DATA_BLOCK DB 99
NAME : OhneName
VERSION : 1.0


 STRUCT
  OFFSET_TABLE: STRUCT
   Offset_Table : STRUCT
    Offset_Type : WORD := W#16#1;
    Offset_Length : WORD := W#16#1E;
    Offset_Address : WORD := W#16#0;
   END_STRUCT ;
   Processdata_Long_Table : STRUCT
    Processdata_Long_Type : WORD := W#16#6;
    Processdata_Long_Length : WORD := W#16#C;
    Processdata_Long_Address : WORD := W#16#1E;
   END_STRUCT ;
   Control_Table : STRUCT
    Control_Type : WORD := W#16#5;
    Control_Length : WORD := W#16#6;
    Control_Address : WORD := W#16#2A;
   END_STRUCT ;
   CAM_MT_Table : STRUCT
    CAM_MT_Type : WORD := W#16#7;
    CAM_MT_Length : WORD := W#16#48;
    CAM_MT_Address : WORD := W#16#30;
   END_STRUCT ;
   AngleTimeCAM_ST_Table : STRUCT
    AT_Cam_ST_Type : WORD := W#16#B;
    AT_Cam_ST_Length : WORD := W#16#6;
    AT_Cam_ST_Address : WORD := W#16#78;
   END_STRUCT ;
  END_STRUCT ;
  Processdata_Long_Table : STRUCT
   Position : DWORD := DW#16#0;
   Speed : WORD := W#16#0;
   Act_Prog : BYTE := B#16#0;
   ErrorNo : BYTE := B#16#0;
   Output1to8 : BYTE := B#16#0;
   Output9to16 : BYTE := B#16#0;
   Output17to24 : BYTE := B#16#0;
   Output25to32 : BYTE := B#16#0;
  END_STRUCT ;
  Control_Table : STRUCT
   New_Prog : BYTE := B#16#0;
   Teach_In_Zero : BOOL := FALSE;
   Invert_Encoder : BOOL := FALSE;
   Error_Quit : BOOL := FALSE;
   Res_03 : BOOL := FALSE;
   Res_04 : BOOL := FALSE;
   Res_05 : BOOL := FALSE;
   Res_06 : BOOL := FALSE;
   Res_07 : BOOL := FALSE;
   Res_0 : BYTE := B#16#0;
   Res_1 : BYTE := B#16#0;
   Res_2 : BYTE := B#16#0;
   Res_3 : BYTE := B#16#0;
  END_STRUCT ;
  CAM_MT_Table : STRUCT
   Cam_MT : ARRAY [ 1 .. 6 ] OF STRUCT
    ProgNo : WORD := W#16#0;
    Output : WORD := W#16#0;
    On : DWORD := DW#16#0;
    Off : DWORD := DW#16#0;
   END_STRUCT ;
  END_STRUCT ;
  AngleTimeCAM_ST_Table : STRUCT
   AT_Cam_ST : ARRAY [ 1 .. 1 ] OF STRUCT
    ProgNo : BYTE := B#16#0;
    Output : BYTE := B#16#0;
    On : WORD := W#16#0;
    Duration : WORD := W#16#0;
   END_STRUCT ;
  END_STRUCT ;
 END_STRUCT ;
BEGIN
   Offset_Table.Offset_Table.Offset_Type := W#16#1;
   Offset_Table.Offset_Table.Offset_Length := W#16#1E;
   Offset_Table.Offset_Table.Offset_Address := W#16#0;
   Offset_Table.Processdata_Long_Table.Processdata_Long_Type := W#16#6;
   Offset_Table.Processdata_Long_Table.Processdata_Long_Length := W#16#C;
   Offset_Table.Processdata_Long_Table.Processdata_Long_Address := W#16#1E;
   Offset_Table.Control_Table.Control_Type := W#16#5;
   Offset_Table.Control_Table.Control_Length := W#16#6;
   Offset_Table.Control_Table.Control_Address := W#16#2A;
   Offset_Table.CAM_MT_Table.CAM_MT_Type := W#16#7;
   Offset_Table.CAM_MT_Table.CAM_MT_Length := W#16#48;
   Offset_Table.CAM_MT_Table.CAM_MT_Address := W#16#30;
   Offset_Table.AngleTimeCAM_ST_Table.AT_Cam_ST_Type := W#16#B;
   Offset_Table.AngleTimeCAM_ST_Table.AT_Cam_ST_Length := W#16#6;
   Offset_Table.AngleTimeCAM_ST_Table.AT_Cam_ST_Address := W#16#78;
   Processdata_Long_Table.Position := DW#16#0;
   Processdata_Long_Table.Speed := W#16#0;
   Processdata_Long_Table.Act_Prog := B#16#0;
   Processdata_Long_Table.ErrorNo := B#16#0;
   Processdata_Long_Table.Output1to8 := B#16#0;
   Processdata_Long_Table.Output9to16 := B#16#0;
   Processdata_Long_Table.Output17to24 := B#16#0;
   Processdata_Long_Table.Output25to32 := B#16#0;
   Control_Table.New_Prog := B#16#0;
   Control_Table.Teach_In_Zero := FALSE;
   Control_Table.Invert_Encoder := FALSE;
   Control_Table.Error_Quit := FALSE;
   Control_Table.Res_03 := FALSE;
   Control_Table.Res_04 := FALSE;
   Control_Table.Res_05 := FALSE;
   Control_Table.Res_06 := FALSE;
   Control_Table.Res_07 := FALSE;
   Control_Table.Res_0 := B#16#0;
   Control_Table.Res_1 := B#16#0;
   Control_Table.Res_2 := B#16#0;
   Control_Table.Res_3 := B#16#0;
   CAM_MT_Table.Cam_MT[1].ProgNo := W#16#0;
   CAM_MT_Table.Cam_MT[1].Output := W#16#0;
   CAM_MT_Table.Cam_MT[1].On := DW#16#0;
   CAM_MT_Table.Cam_MT[1].Off := DW#16#0;
   CAM_MT_Table.Cam_MT[2].ProgNo := W#16#0;
   CAM_MT_Table.Cam_MT[2].Output := W#16#0;
   CAM_MT_Table.Cam_MT[2].On := DW#16#0;
   CAM_MT_Table.Cam_MT[2].Off := DW#16#0;
   CAM_MT_Table.Cam_MT[3].ProgNo := W#16#0;
   CAM_MT_Table.Cam_MT[3].Output := W#16#0;
   CAM_MT_Table.Cam_MT[3].On := DW#16#0;
   CAM_MT_Table.Cam_MT[3].Off := DW#16#0;
   CAM_MT_Table.Cam_MT[4].ProgNo := W#16#0;
   CAM_MT_Table.Cam_MT[4].Output := W#16#0;
   CAM_MT_Table.Cam_MT[4].On := DW#16#0;
   CAM_MT_Table.Cam_MT[4].Off := DW#16#0;
   CAM_MT_Table.Cam_MT[5].ProgNo := W#16#0;
   CAM_MT_Table.Cam_MT[5].Output := W#16#0;
   CAM_MT_Table.Cam_MT[5].On := DW#16#0;
   CAM_MT_Table.Cam_MT[5].Off := DW#16#0;
   CAM_MT_Table.Cam_MT[6].ProgNo := W#16#0;
   CAM_MT_Table.Cam_MT[6].Output := W#16#0;
   CAM_MT_Table.Cam_MT[6].On := DW#16#0;
   CAM_MT_Table.Cam_MT[6].Off := DW#16#0;
   AngleTimeCAM_ST_Table.AT_Cam_ST[1].ProgNo := B#16#0;
   AngleTimeCAM_ST_Table.AT_Cam_ST[1].Output := B#16#0;
   AngleTimeCAM_ST_Table.AT_Cam_ST[1].On := W#16#0;
   AngleTimeCAM_ST_Table.AT_Cam_ST[1].Duration := W#16#0;
END_DATA_BLOCK
